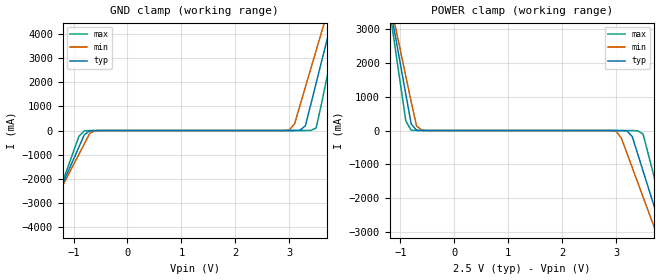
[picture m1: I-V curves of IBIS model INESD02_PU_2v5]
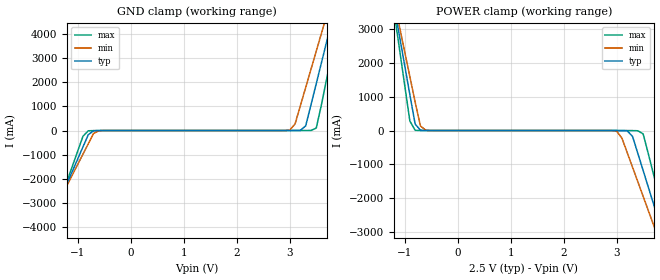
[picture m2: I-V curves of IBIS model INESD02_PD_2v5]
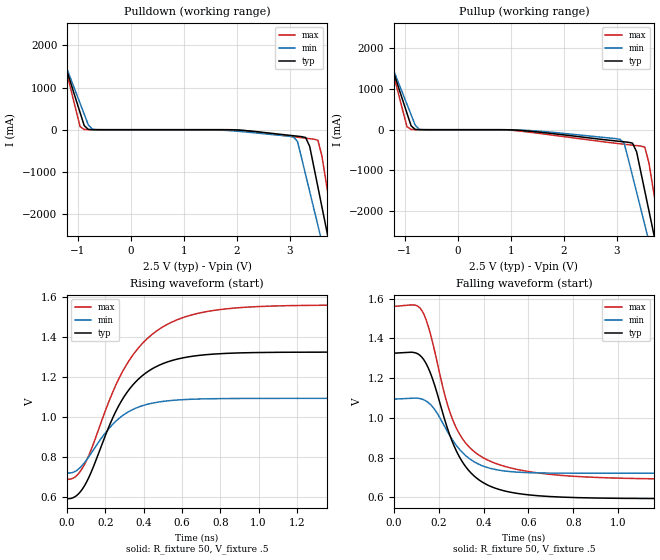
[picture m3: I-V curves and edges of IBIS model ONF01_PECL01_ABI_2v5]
|   This file is an IBIS representation of the   |
|   Integrated Devices Technology, Inc.   |
|   ICS813001I   |
|   DUAL VCXO W/3.3V, 2.5V LVPECL  FEMTOCLOCK PLL   |
[IBIS Ver]   4.1
[File name]   813001i.ibs
[File Rev]   1.0
[Date]   13 Jan 2009 | Last modified
|   24 Dec 2008 | Generated
[Source]   Originated at Integrated Devices Technology, Inc.
[Disclaimer]
IDT hereby grants the user of this IBIS model a non-exclusive,
nontransferable license to use this IBIS model under the following terms.
Before using this IBIS model, the user should read this license.
If the user does not accept these terms,  the IBIS model should be
returned to IDT within 30 days.
   The user is granted this license only to use the IBIS model and
is not granted rights to sell, load, rent, lease or license the IBIS
model in whole or in part, or in modified form to anyone other than
user. User may modify the IBIS model to suit its specific
applications but rights to derivative works and such modifications
shall belong to IDT.
   This IBIS model is provided on an "AS IS" basis and IDT makes
absolutely no warranty with respect to the information contained
herein. IDT DISCLAIMS AND CUSTOMER WAIVES ALL WARRANTIES, EXPRESS
OR IMPLIED, INCLUDING WARRANTIES OF MERCHANTABILITY OR FITNESS FOR
A PARTICULAR PURPOSE. The entire risk as to quality and performance
is with the Customer. ACCORDINGLY, IN NO EVENT SHALL THE COMPANY BE
LIABLE FOR ANY DAMAGES, WHETHER IN CONTRACT OR TORT,INCLUDING ANY
LOST PROFITS OR OTHER INCIDENTAL, CONSEQUENTIAL, EXEMPLARY, OR
PUNITIVE DAMAGES ARISING OUT OF THE USE OR APPLICATION OF THE IBIS
model provided in this package. Further, IDT reserves the right to
make changes without notice to any product herein to improve
reliability, function, or design. IDT does not convey any license
under patent rights or any other intellectual property rights,
including those of third parties.
   IDT is not obligated to provide maintenance or support
for the licensed IBIS model.
[Copyright]   Copyright 2004 byIntegrated Devices Technology, Inc.
[Component]   ICS813001GI
[Manufacturer] Integrated Devices Technology, Inc.
[Package]
|TSSOP 24 Lead
|   typ   min   max
R_pkg   60.65m   52.4m   68.9m
L_pkg   1.989nH   1.431nH   2.547nH
C_pkg   0.314pF   0.254pF   0.374pF
[Pin]   signal_name   model_name   R_pin   L_pin   C_pin
1   VCO_SEL   INESD02_PU   68.9m   2.547n   0.374p
2   N0   INESD02_PU   65.6m   2.323n   0.350p
3   N1   INESD02_PU   62.3m   2.100n   0.326p
4   N2   INESD02_PD   59.0m   1.877n   0.302p
5   VCCO   POWER   55.7m   1.654n   0.278p
6   Q   ONF01_PECL01_ABI   52.4m   1.431n   0.254p
7   nQ   ONF01_PECL01_ABI   52.4m   1.431n   0.254p
8   VEE   GND   55.7m   1.654n   0.278p
9   VCCA   POWER   59.0m   1.877n   0.302p
10   VCC   POWER   62.3m   2.100n   0.326p
11   XTAL_OUT1   NC   65.6m   2.323n   0.350p
12   XTAL_IN1   NC   68.9m   2.547n   0.374p
13   XTAL_OUT0   NC   68.9m   2.547n   0.374p
14   XTAL_IN0   NC   65.6m   2.323n   0.350p
15   VC   NC   62.3m   2.100n   0.326p
16   CLK0   INESD02_PD_PECL   59.0m   1.877n   0.302p
17   nCLK1   INESD02_PU_PECL   55.7m   1.654n   0.278p
18   CLK1   INESD02_PD_PECL   52.4m   1.431n   0.254p
19   MO   INESD02_PU   52.4m   1.431n   0.254p
20   M1   INESD02_PD   55.7m   1.654n   0.278p
21   M2   INESD02_PD   59.0m   1.877n   0.302p
22   OE   INESD02_PU   62.3m   2.100n   0.326p
23   CLK_SEL1   INESD02_PU   65.6m   2.323n   0.350p
24   CLK_SEL0   INESD02_PD   68.9m   2.547n   0.374p
[Diff Pin]  inv_pin  vdiff tdelay_typ tdelay_min  tdelay_max
18   17   0.15   0   0   0
6   7   NA   0   0   0
[Model Selector] INESD02_PU
INESD02_PU_2v5  Buffer selection for 2v5
INESD02_PU_3v3  Buffer selection for 3v3
[Model Selector] INESD02_PD
INESD02_PD_2v5  Buffer selection for 2v5
INESD02_PD_3v3  Buffer selection for 3v3
[Model Selector] ONF01_PECL01_ABI
ONF01_PECL01_ABI_2v5  Buffer selection for 2v5
ONF01_PECL01_ABI_3v3  Buffer selection for 3v3
[Model Selector] INESD02_PD_PECL
INESD02_PD_PECL_2v5  Buffer selection for 2v5
INESD02_PD_PECL_3v3  Buffer selection for 3v3
[Model Selector] INESD02_PU_PECL
INESD02_PU_PECL_2v5  Buffer selection for 2v5
INESD02_PU_PECL_3v3  Buffer selection for 3v3
| Models and submodels in the file (10): INESD02_PU_2v5 (Input), INESD02_PD_2v5 (Input), ONF01_PECL01_ABI_2v5 (Output_ECL), INESD02_PD_PECL_2v5 (Input), INESD02_PU_PECL_2v5 (Input), INESD02_PU_3v3 (Input), INESD02_PD_3v3 (Input), ONF01_PECL01_ABI_3v3 (Output_ECL), INESD02_PD_PECL_3v3 (Input), INESD02_PU_PECL_3v3 (Input)
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[Model] INESD02_PU_2v5
Model_type   Input
Polarity   Non-Inverting
Vinl = 1.4V
Vinh = 1.85V
|   typ   min   max
C_comp   2pF   1.5pF   2.5pF
|   typ   min   max
[Voltage range]  2.5V   2.375V   2.625V
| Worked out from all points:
|   GND clamp passes 1 mA (typ) near -0.55 V on its own axis
|   POWER clamp passes 1 mA (typ) near -0.61 V on its own axis
[GND_clamp]
|Voltage   I(typ)   I(min)   I(max)
-2.5V     -8.775A    -7.892A    -10.18A
-1.6V     -4.218A    -4.001A    -4.586A
-900mV    -678.5mA   -979.4mA   -237.6mA
-800mV    -173.9mA   -548.7mA   -10.88mA
-600mV    -1.682mA   -8.796mA   -960.5uA
3V        79.39uA    17.1mA     7.198uA
3.1V      607uA      273.4mA    11.46uA
3.3V      191.5mA    1.785A     278.5uA
3.5V      1.949A     3.298A     103.5mA
3.7V      3.723A     4.812A     2.189A
3.9V      5.498A     6.327A     4.369A
5V        15.27A     14.67A     16.38A
[POWER_clamp]
|Voltage   I(typ)   I(min)   I(max)
-2.5V     15.27A     13.72A     17.74A
-1.2V     3.723A     3.866A     3.551A
-1.1V     2.836A     3.109A     2.461A
-900mV    1.063A     1.596A     283.3mA
-800mV    191.5mA    840mA      6.139mA
-600mV    607uA      8.789mA    64.82uA
3V        -392uA     -16.42mA   -62.09uA
3.4V      -678.5mA   -1.518A    -7.233mA
3.5V      -1.184A    -1.95A     -99.57mA
3.7V      -2.195A    -2.813A    -1.324A
4V        -3.712A    -4.109A    -3.188A
5V        -8.775A    -8.433A    -9.404A
[Model] INESD02_PD_2v5
Model_type   Input
Polarity   Non-Inverting
Vinl = 1.4V
Vinh = 1.85V
|   typ   min   max
C_comp   2pF   1.5pF   2.5pF
|   typ   min   max
[Voltage range]  2.5V   2.375V   2.625V
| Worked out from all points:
|   GND clamp passes 1 mA (typ) near -0.55 V on its own axis
|   POWER clamp passes 1 mA (typ) near -0.60 V on its own axis
[GND_clamp]
|Voltage I(typ)   I(min)   I(max)
-2.5V     -8.775A    -7.892A    -10.18A
-1.6V     -4.218A    -4.001A    -4.586A
-900mV    -678.5mA   -979.3mA   -237.6mA
-800mV    -173.9mA   -548.7mA   -10.83mA
-600mV    -1.629mA   -8.74mA    -911.1uA
3V        133.3uA    17.16mA    56.6uA
3.1V      660.9uA    273.5mA    60.87uA
3.3V      191.6mA    1.785A     327.9uA
3.5V      1.949A     3.298A     103.6mA
3.7V      3.723A     4.812A     2.189A
3.9V      5.498A     6.327A     4.369A
5V        15.27A     14.67A     16.38A
[POWER_clamp]
|Voltage   I(typ)   I(min)   I(max)
-2.5V     15.27A     13.72A     17.74A
-1.2V     3.723A     3.866A     3.551A
-1.1V     2.836A     3.109A     2.461A
-900mV    1.063A     1.596A     283.3mA
-800mV    191.6mA    840.1mA    6.189mA
-600mV    660.9uA    8.845mA    114.2uA
3V        -338.1uA   -16.36mA   -12.68uA
3.4V      -678.5mA   -1.518A    -7.183mA
3.5V      -1.183A    -1.95A     -99.52mA
3.7V      -2.195A    -2.813A    -1.324A
4V        -3.712A    -4.109A    -3.188A
5V        -8.775A    -8.432A    -9.404A
[Model] ONF01_PECL01_ABI_2v5
Model_type  Output_ECL
Polarity   Non-Inverting
Vmeas = .975
Rref = 50
Cref = 0
Vref = .5
|Variable  typ   min   max
C_comp   2p   1.5p   2.5p
[Voltage Range]   2.5   2.375   2.625
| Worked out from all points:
|   rising waveform, R_fixture 50, V_fixture .5: 20-80 % time 228ps typ, 199ps min, 276ps max; typ from 0.592 V to 1.33 V
|   falling waveform, R_fixture 50, V_fixture .5: 20-80 % time 153ps typ, 140ps min, 156ps max; typ from 1.33 V to 0.592 V
| Open source, no load
|  Voltage   I(typ)   I(min)   I(max)
[Pullup]
-2.5V     6.581A     5.758A     7.966A
-1.572V   2.868A     2.671A     3.219A
-1.418V   2.25A      2.158A     2.429A
-953.6mV  402.1mA    621.9mA    72.14mA
-876.3mV  95.6mA     366.6mA    5.897mA
-721.6mV  951.4uA    9.59mA     751.4uA
3.067V    -287.8mA   -237.7mA   -346mA
3.299V    -330.4mA   -1.134A    -380.1mA
3.531V    -1.506A    -2.34A     -427.9mA
3.686V    -2.47A     -3.144A    -1.427A
3.84V     -3.434A    -3.947A    -2.655A
5V        -10.66A    -9.976A    -11.86A
[Pulldown]
-2.5V     6.581A     5.758A     7.966A
-1.495V   2.559A     2.415A     2.824A
-1.418V   2.25A      2.158A     2.429A
-953.6mV  402.1mA    621.9mA    72.14mA
-876.3mV  95.6mA     366.6mA    5.897mA
-721.6mV  951.4uA    9.59mA     751.4uA
3.067V    -142.9mA   -171.4mA   -166.7mA
3.299V    -185mA     -1.067A    -201.5mA
3.531V    -1.361A    -2.272A    -250mA
3.686V    -2.324A    -3.076A    -1.249A
3.84V     -3.288A    -3.879A    -2.478A
5V        -10.51A    -9.904A    -11.69A
[Ramp]
|   typ   min   max
dV/dt_r   0.586/0.368n   0.299/0.313n   0.698/0.446n
dV/dt_f   0.590/0.258n   0.302/0.226n   0.703/0.290n
R_load =   50.0000
[Rising Waveform]
R_fixture = 50
V_fixture = .5   | VCC_typ - 2V
V_fixture_max = 0.625   | VCC_max - 2V
V_fixture_min = 0.375   | VCC_min - 2V
C_fixture = 0.0p
| Time   typ   min   max
0s        592.5mV    720.8mV    689.3mV
46.2ps    605.5mV    731.1mV    704.8mV
92.4ps    659.4mV    774.5mV    766.4mV
241.5ps   1.003V     967.6mV    1.133V
323.4ps   1.138V     1.029V     1.283V
426.3ps   1.231V     1.066V     1.4V
552.3ps   1.285V     1.084V     1.478V
711.9ps   1.312V     1.092V     1.525V
940.8ps   1.323V     1.094V     1.551V
1.999ns   1.326V     1.094V     1.562V
[Falling Waveform]
R_fixture = 50
V_fixture = .5   | VCC_typ - 2V
V_fixture_max = 0.625   | VCC_max - 2V
V_fixture_min = 0.375   | VCC_min - 2V
C_fixture = 0.0p
| Time   typ   min   max
0s        1.326V     1.094V     1.562V
92.4ps    1.328V     1.099V     1.568V
123.9ps   1.306V     1.095V     1.541V
168ps     1.209V     1.061V     1.4V
231ps     973.8mV    945.4mV    1.097V
277.2ps   835.9mV    862.7mV    951mV
348.6ps   716.5mV    784.8mV    838.7mV
447.3ps   647.2mV    740.6mV    773mV
865.2ps   596.5mV    720.8mV    701.4mV
1.999ns   592.4mV    720.7mV    689.3mV
